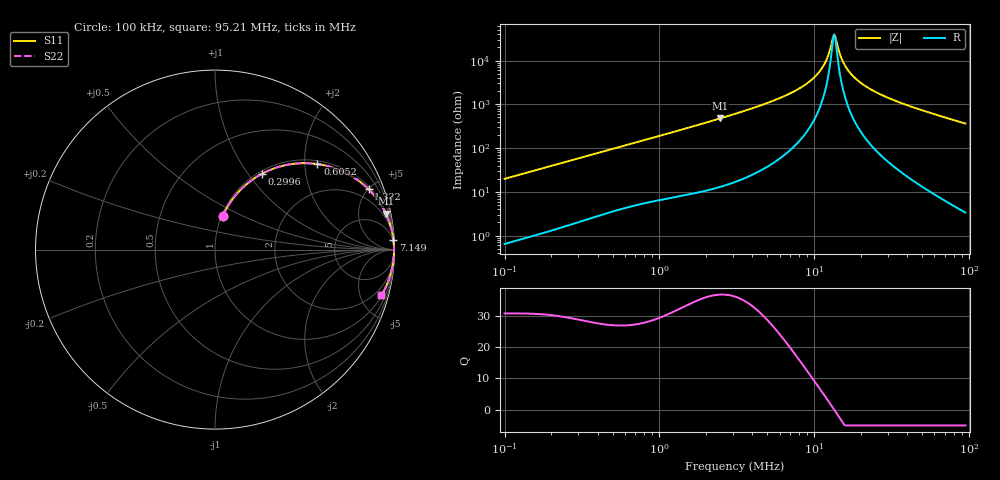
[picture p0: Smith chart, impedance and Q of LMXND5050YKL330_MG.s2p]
! LMXND5050YKL330_MG  S-PARAMETER MODEL  ( General Type )
! Model Generated by TAIYO YUDEN Corporation (https://www.yuden.co.jp/en/)
! Version 1.0
! TAIYO YUDEN Control No. 191023NI43SB-FBB
! Copyright(c) 2019 TAIYO YUDEN CO.,LTD. All Rights Reserved.
! Product Description (link to TY-COMPAS)
! https://ds.yuden.co.jp/TYCOMPAS/or/detail?pn=LMXND5050YKL330MMG&u=M
! Products Name : Inductors
! Characteristics :
!  Inductance : 33 uH , SRF(min) : 7.0 MHz , DC Resistance(max) : 0.234 Ohm
!  Rated Current : Saturation :1300 mA , Temp Rise : 1200 mA (40 degC)
!  Case Size : 4.9 x 4.9 / 0.193 x 0.193 [mm/inch] , Thickness : 4 / 0.157 [mm/inch]
!  (Conditions: Temperature = 25 degC , DC Bias Current/Voltage = 0A / 0V)
! External Node Assignments :
!  1  o---GGG---o  2
! GND o---------o GND
! Frequency Range : 0.1MHz  -  95.211795MHz  [ 402 STEP ]
# MHz S RI R 50
! Freq[MHz].  S11 Real  S11 Imag  S21 Real  S21 Imag  S12 Real  S12 Imag  S22 Real  S22 Imag
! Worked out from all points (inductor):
!   401 points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, 100 kHz to 95.21 MHz, reference 50 ohm
!   read as one part in series: L = 31.4 uH near 103.5 kHz
!   highest Q = 36.7 at 2.469 MHz (marker M1), where L = 30.6 uH
!   self-resonance near 13.48 MHz
!   S11 on the Smith chart (normalised r, x): 100 kHz: 1.01, +0.40; 299.6 kHz: 1.04, +1.17; 605.2 kHz: 1.09, +2.31; 1.332 MHz: 1.16, +5.03; 7.149 MHz: 3, +37; 95.21 MHz: 1.07, -7.26
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0.1  0.0436 0.1886  0.9564 -0.1886  0.9564 -0.1886  0.0436 0.1886
0.179138  0.1182 0.3068  0.8818 -0.3068  0.8818 -0.3068  0.1182 0.3068
0.299634  0.2611 0.4221  0.7389 -0.4221  0.7389 -0.4221  0.2611 0.4221
0.31545  0.2802 0.4319  0.7198 -0.4319  0.7198 -0.4319  0.2802 0.4319
0.60521  0.5702 0.4768  0.4298 -0.4768  0.4298 -0.4768  0.5702 0.4768
0.995088  0.7725 0.4024  0.2275 -0.4024  0.2275 -0.4024  0.7725 0.4024
1.331851  0.8561 0.3357  0.1439 -0.3357  0.1439 -0.3357  0.8561 0.3357
2.469096  0.9525 0.1994  0.0475 -0.1994  0.0475 -0.1994  0.9525 0.1994
3.085641  0.9691 0.1596  0.0309 -0.1596  0.0309 -0.1596  0.9691 0.1596
7.14883  0.9943 0.0539  0.00575 -0.0539  0.00575 -0.0539  0.9943 0.0539
9.733658  0.9967 0.0266  0.00334 -0.0266  0.00334 -0.0266  0.9967 0.0266
11.55429  0.9973 0.0125  0.00272 -0.0125  0.00272 -0.0125  0.9973 0.0125
12.37457  0.9974 0.00705  0.0026 -0.00705  0.0026 -0.00705  0.9974 0.00705
13.25309  0.9975 0.00159  0.00253 -0.00159  0.00253 -0.00159  0.9975 0.00159
13.4823  0.9975 0.00023  0.00253 -0.00023  0.00253 -0.00023  0.9975 0.00023
13.95267  0.9975 -0.00249  0.00252 0.00249  0.00252 0.00249  0.9975 -0.00249
14.68918  0.9974 -0.00659  0.00255 0.00659  0.00255 0.00659  0.9974 -0.00659
15.46457  0.9974 -0.0107  0.00261 0.0107  0.00261 0.0107  0.9974 -0.0107
17.73828  0.997 -0.0218  0.00295 0.0218  0.00295 0.0218  0.997 -0.0218
22.16762  0.9959 -0.0408  0.00413 0.0408  0.00413 0.0408  0.9959 -0.0408
30.70484  0.9923 -0.0723  0.00772 0.0723  0.00772 0.0723  0.9923 -0.0723
95.21179  0.9274 -0.2548  0.0726 0.2548  0.0726 0.2548  0.9274 -0.2548
